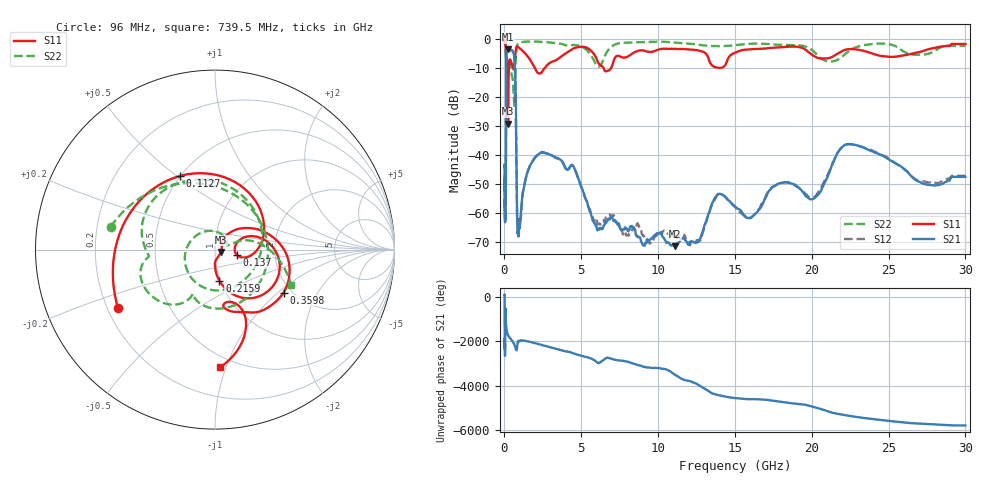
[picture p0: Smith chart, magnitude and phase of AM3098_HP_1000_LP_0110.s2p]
! Date/Time: Thu, Feb 28, 2019 8:39 AM
! Network Analyzer: Agilent Technologies E8364B Rev: A.07.50.67
! Sweep from 0.010 to 30.000 GHz, 1601 Points, Sweep Type: LOG
! Power Supply: 5.022 V, 0.002 A
# Hz S DB R 50
!freq MagS11 AngS11 MagS21 AngS21 MagS12 AngS12 MagS22 AngS22
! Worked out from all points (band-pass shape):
!   1601 points, 10 MHz to 30 GHz, reference 50 ohm
!   highest |S21| = -3.38 dB at 236.3 MHz (marker M1); lowest = -71.6 dB at 11.08 GHz (marker M2)
!   |S21| within 3 dB of the highest: 127.3 MHz to 643.8 MHz (516.5 MHz wide, 134 % of centre)
!   lowest |S11| = -29.2 dB at 236.3 MHz (marker M3), VSWR 1.07, Z = 53.3 - j1.34 ohm
!   |S11| at or under -10 dB: 198.7 MHz to 287.3 MHz (88.58 MHz wide, 36.4 % of centre); 1.991 GHz to 2.602 GHz (610.8 MHz wide, 26.6 % of centre); 6.455 GHz to 6.931 GHz (476.7 MHz wide, 7.12 % of centre)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
!   |S22| runs from -23.0 to -0.6 dB; largest |S21 - S12| = 0.012
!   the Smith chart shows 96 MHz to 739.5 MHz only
!   S11 on the Smith chart (normalised r, x): 96 MHz: 0.24, -0.26; 112.7 MHz: 0.50, +0.51; 137 MHz: 1.28, -0.08; 215.9 MHz: 0.99, -0.35; 359.8 MHz: 1.82, -1.09; 739.5 MHz: 0.42, -0.96
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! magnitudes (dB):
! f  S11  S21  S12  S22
! 10 MHz  -0.4  -44.0  -44.1  -0.6
! 38.04 MHz  -0.5  -61.8  -62.1  -0.8
! 86.86 MHz  -2.8  -54.6  -51.5  -3.0
! 96 MHz  -4.0  -41.1  -41.1  -4.5
! 112.7 MHz  -6.9  -16.4  -16.4  -10.5
! 137 MHz  -17.9  -4.8  -4.8  -11.2
! 144.7 MHz  -18.5  -4.4  -4.3  -10.5
! 215.9 MHz  -15.1  -3.5  -3.5  -8.2
! 236.3 MHz  -29.2  -3.4  -3.4  -8.6
! 359.8 MHz  -6.9  -3.8  -3.8  -7.7
! 550.5 MHz  -9.7  -4.3  -4.2  -14.6
! 646.1 MHz  -9.6  -6.5  -6.5  -22.9
! 739.5 MHz  -3.7  -24.2  -24.2  -6.6
! 821.5 MHz  -2.4  -60.9  -59.9  -2.2
! 894.4 MHz  -2.7  -67.5  -65.2  -1.4
! 2.084 GHz  -11.0  -40.3  -40.5  -0.8
! 4.436 GHz  -3.3  -43.8  -43.5  -1.9
! 7.926 GHz  -6.2  -65.4  -67.9  -1.1
! 11.08 GHz  -3.3  -71.6  -67.4  -1.1
! 20.1 GHz  -5.6  -55.2  -54.7  -4.1
! 22.56 GHz  -3.4  -36.3  -36.2  -3.5
! 30 GHz  -1.6  -47.6  -47.2  -2.3
